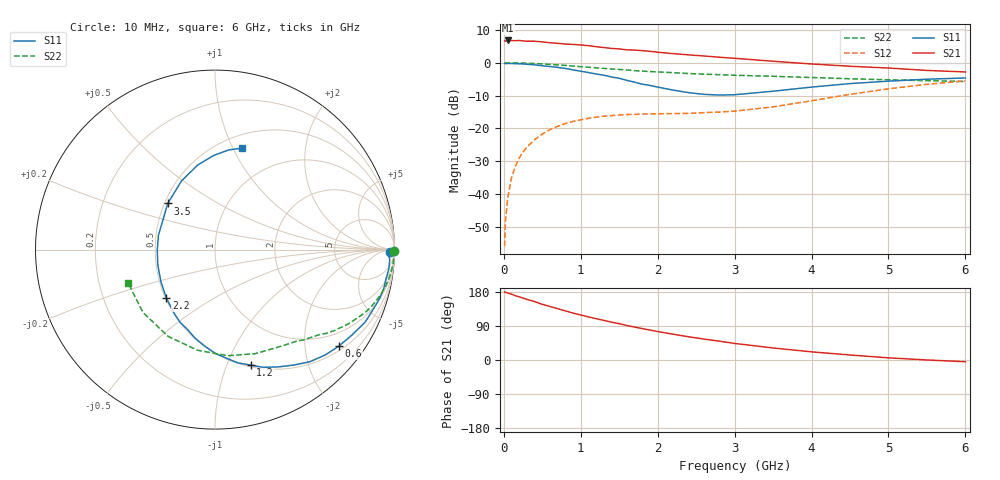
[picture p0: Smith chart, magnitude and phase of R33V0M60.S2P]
! SIEMENS Small Signal Semiconductors
! BFR181
! Si NPN RF Bipolar Junction Transistor in SOT23
! VCE = 3 V  IC = 0.6 mA
! Common Emitter S-Parameters:  May  1996
# GHz  S  MA  R  50
!  f  S11  S21  S12  S22
! GHz  MAG  ANG  MAG  ANG  MAG  ANG  MAG  ANG
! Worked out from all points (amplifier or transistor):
!   36 points, 10 MHz to 6 GHz, reference 50 ohm
!   highest |S21| = 6.8 dB at 50 MHz (marker M1)
!   |S21| within 3 dB of that: start of sweep to 1.74 GHz
!   unconditionally stable (mu >= 1): 2.268 GHz to 3.878 GHz
!   at 250 MHz: K = 0.13, MSG = 16.9 dB, |S12| = -27.2 dB
!   at 1.4 GHz: K = 0.64, MSG = 10.2 dB, |S12| = -16.1 dB
!   at 6 GHz: K = 0.91, MSG = 1.4 dB, |S12| = -5.5 dB
!   S11 on the Smith chart (normalised r, x): 10 MHz: 68, -37; 600 MHz: 0.61, -2.79; 1.2 GHz: 0.52, -1.22; 2.2 GHz: 0.51, -0.32; 3.5 GHz: 0.52, +0.31; 6 GHz: 0.63, +1.09
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0.01  0.9775 -0.7  2.158 179.7  0.0016 89.1  0.9989 -0.3
0.02  0.9663 -1.2  2.119 178.6  0.0037 91.2  0.9957 -0.6
0.05  0.975 -3.3  2.185 176.8  0.0086 88.3  0.9985 -1.5
0.1  0.9746 -6.4  2.177 173.8  0.0177 85.3  0.9964 -3.1
0.2  0.9649 -12.9  2.184 166.6  0.0352 81.2  0.9916 -6.1
0.3  0.9471 -19.2  2.125 159.9  0.0519 76.7  0.9838 -9.0
0.4  0.9292 -25.8  2.126 154.2  0.0672 72.7  0.9726 -12.0
0.5  0.8986 -32.1  2.078 146.8  0.0819 68.6  0.9584 -14.8
0.6  0.8748 -38.0  2.014 141.3  0.0957 64.5  0.9435 -17.4
0.9  0.7782 -55.8  1.901 123.7  0.1277 54.2  0.89 -24.6
1.1  0.7084 -67.8  1.818 113.8  0.1422 48.7  0.8535 -28.7
1.2  0.6736 -72.8  1.755 109.1  0.148 46.1  0.8356 -30.7
1.7  0.5051 -102.8  1.56 86.9  0.163 38.4  0.7571 -38.4
2  0.4257 -121.6  1.445 75.1  0.167 36.5  0.7244 -42.5
2.2  0.3827 -135.0  1.377 68.1  0.1678 36.4  0.7052 -45.5
2.6  0.3298 -165.2  1.267 55.3  0.1735 39.1  0.6701 -51.0
3  0.3251 165.6  1.168 43.7  0.1829 43.4  0.644 -58.0
3.5  0.3679 135.7  1.054 31.8  0.2123 48.6  0.6215 -68.9
4  0.4252 116.1  0.957 21.5  0.2633 51.2  0.5956 -83.0
4.5  0.4809 101.6  0.884 13.2  0.3297 49.1  0.5694 -99.8
5.5  0.5609 82.1  0.763 0.1  0.4688 36.6  0.5327 -138.9
6  0.5855 74.9  0.723 -4.6  0.5287 28.0  0.5185 -159.0
